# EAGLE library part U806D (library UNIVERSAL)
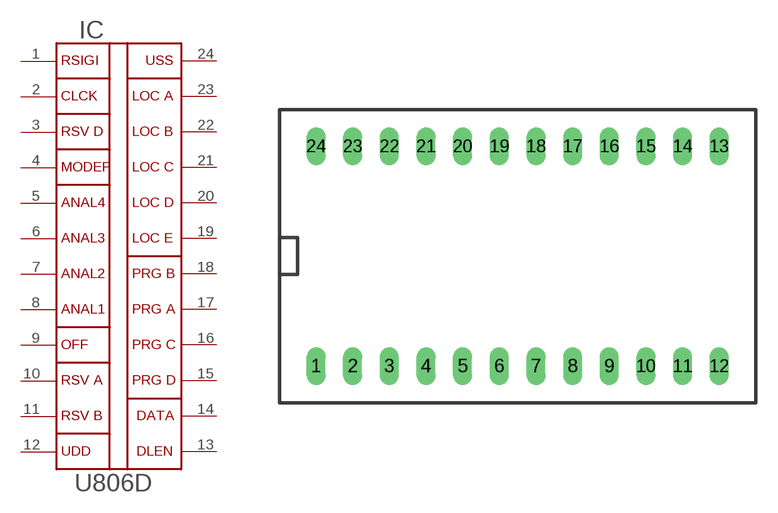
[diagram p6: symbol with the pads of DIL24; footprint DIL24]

Designator prefix IC

## U806D  [DIL24]
1  P$1
2  P$2
3  P$3
4  P$4
5  P$5
6  P$6
7  P$7
8  P$8
9  P$9
10  P$10
11  P$11
12  P$12
13  P$13
14  P$14
15  P$15
16  P$16
17  P$17
18  P$18
19  P$19
20  P$20
21  P$21
22  P$22
23  P$23
24  P$24

## Footprint DIL24 (pad centres in mm)
drill 0.813 pad 1.092 long: 1 0,0; 2 2.54,0; 3 5.08,0; 4 7.62,0; 5 10.16,0; 6 12.7,0; 7 15.24,0; 8 17.78,0; 9 20.32,0; 10 22.86,0; 11 25.4,0; 12 27.94,0; 13 27.94,15.24; 14 25.4,15.24; 15 22.86,15.24; 16 20.32,15.24; 17 17.78,15.24; 18 15.24,15.24; 19 12.7,15.24; 20 10.16,15.24; 21 7.62,15.24; 22 5.08,15.24; 23 2.54,15.24; 24 0,15.24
